// ***************************************************************************
// UDT985

// Datum	  Name	Aktion
// ---------------------------------------------------------------------------
// 29.10.97   Mahler	Neu

TYPE "XC_JOB_SR_UDT"	// User-Auftrag fuer Send/Receive Schnittstelle

STRUCT

	iPCU			: INT;				//0: inaktiv

	bType			: BYTE	:= B#16#E;		//Auftrags-Typ
									//14=GET, 15=PUT, 16=PUT_Time

	boEnable		: BOOL;				//1: Auftrag freigegeben
	boParamError	: BOOL;				//Auftragsparameter fehlerhaft
	boPCU_Error		: BOOL;				//PCU in STOP oder Verb.fehler
	bo3			: BOOL;
	boTms			: BOOL;				//TimeBase = 100 ms
	boTmin		: BOOL;				//TimeBase = min           Tms+Tmin=0 dh. TimeBase = sec
	boQuit		: BOOL;				//Auftrag mit Quittung vom Partner
	boTmpJob		: BOOL;				//einmaliger Job, danach PCU:=0, Enable:=0

	bSrc_DType		: BYTE	:= B#16#2;		//Datentyp, 2=byte, 4=word,...
	bSrc_AREA		: BYTE	:= B#16#84;		//0x80..0x84 = P,E,A,M,DB
	iSrc_DB		: INT		:= 200;		//DB-Nummer
	dwSrcByte		: DWORD;
	bSrcBit		: BYTE;
	iSrc_Num		: INT		:= 400;		//Anzahl Bytes 2,4,6,..400

	bDest_DType		: BYTE	:= B#16#2;		//Datentyp, 2=byte, 4=word,...
	bDest_AREA		: BYTE	:= B#16#84;		//0x80..0x84 = P,E,A,M,DB
	iDest_DB		: INT		:= 200;		//DB-Nummer
	dwDestByte		: DWORD;
	bDestBit		: BYTE;
	iDest_Num		: INT		:= 400;		//Anzahl Bytes 2,4,6,..400

	iTime			: INT		:= 10;		//Sollzeit (s)
	iActTime		: INT;				//Istzeit

	iPCU_STATUS	: INT;					//Var. LOCAL v. STATUS (Zustand der Partner-PCU)
									//-2 : TIMEOUT (SISTAR)
									//-1 : Fehler v. STATUS gemeldet (SISTAR)
									//0	: CPU in STOP
									//2	: CPU in RUN
									//weitere siehe Ref.handbuch

	iJobState		: INT;				//Auftragszustand:
									//0=Ruhe, 2=läuft, 4=foF, 8=fmF

	iGetPutStatus	: INT;				//-2 : TIMEOUT (SISTAR)
									//-1 : CPU in STOP (SISTAR)
									//1..20 (SFB 14/15: siehe Ref.handbuch)

	//Ersatzwerte nur bei GET-Auftrag!

	iFltTime		: INT		:= 120;		//Sollzeit
	iFltActTime		: INT		:= 120;		//Istzeit

	bFltSrc_DType	: BYTE	:= B#16#2;		//Datentyp, 2=byte, 4=word,...
	bFltSrc_AREA	: BYTE;				//0: keine Ersatzwerte
									//0x80..0x84 = P,E,A,M,DB
	iFltSrc_DB		: INT		:= 201;		//DB-Nummer
	dwFltSrcByte	: DWORD;
	bFltSrcBit		: BYTE;
	iFltSrc_Num		: INT		:= 400;		//Anzahl Bytes 2,4,6,..400
	iBLKMOV_RET_VAL	: INT;

END_STRUCT ;

END_TYPE


